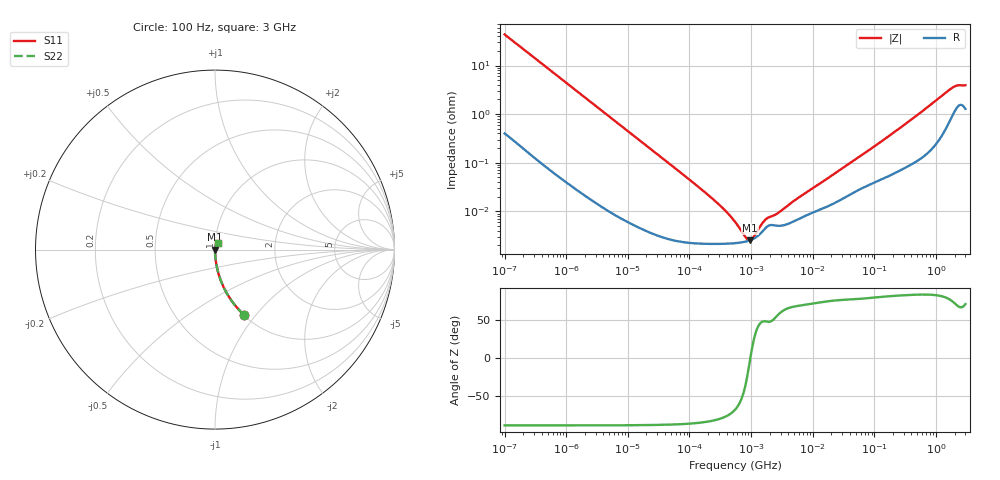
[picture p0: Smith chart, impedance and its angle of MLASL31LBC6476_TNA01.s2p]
! MLASL31LBC6476_TNA01  S-PARAMETER MODEL  ( Standard Model )
! Model Generated by TAIYO YUDEN Corporation (http://www.ty-top.com)
! Version 1.0
! TAIYO YUDEN Control No. 220601
! Copyright(c) 2018 TAIYO YUDEN CO.,LTD. All Rights Reserved.
! Product Description (link to TY-COMPAS)
! https://ds.yuden.co.jp/TYCOMPAS/or/detail?pn=MLASL31LBC6476MTNA01&u=M
! Products Name : Multilayer Ceramic Capacitors
! Characteristics :
!  Capacitance : 47 [uF] , Rated Voltage : 10 [V] , TCC : X6S
!  Case Size : 3.2 x 1.6 / 0.126 x 0.063 [mm/inch] , Thickness : 1.6 / 0.063 [mm/inch]
!  (Conditions: Temperature = 25 [degC] , DC Bias Voltage = 0 [V])
! External Node Assignments :
!  1  o---| |---o  2
! GND o---------o GND
! Frequency Range : 100Hz  -  3GHz  [ 401 STEP ]
# MHZ S RI R 50
! Freq[MHz].  S11 Real  S11 Imag  S21 Real  S21 Imag  S12 Real  S12 Imag  S22 Real  S22 Imag
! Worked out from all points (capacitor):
!   401 points, 100 Hz to 3 GHz, reference 50 ohm
!   read as one part in series: C = 36.5 uF near 109 Hz
!   lowest |Z| = 2.54 mohm at 958.4 kHz (marker M1)
!   series resonance near 973.7 kHz, so ESL is about 730 pH
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0.0001  0.1616 -0.3636  0.8384 0.3636  0.8384 0.3636  0.1616 -0.3636
0.000114  0.1302 -0.332  0.8698 0.332  0.8698 0.332  0.1302 -0.332
0.000175  0.0606 -0.2341  0.9394 0.2341  0.9394 0.2341  0.0606 -0.2341
0.000348  0.0167 -0.1237  0.9833 0.1237  0.9833 0.1237  0.0167 -0.1237
0.000724  0.00421 -0.0605  0.9958 0.0605  0.9958 0.0605  0.00421 -0.0605
0.001788  0.000844 -0.0247  0.9992 0.0247  0.9992 0.0247  0.000844 -0.0247
0.031977  3.28e-05 -0.00141  1 0.00141  1 0.00141  3.28e-05 -0.00141
0.16412  2.16e-05 -0.000268  1 0.000268  1 0.000268  2.16e-05 -0.000268
0.371814  2.15e-05 -0.000104  1 0.000104  1 0.000104  2.15e-05 -0.000104
0.423062  2.16e-05 -8.71e-05  1 8.71e-05  1 8.71e-05  2.16e-05 -8.71e-05
0.547723  2.21e-05 -5.69e-05  1 5.69e-05  1 5.69e-05  2.21e-05 -5.69e-05
0.958445  2.53e-05 -1.48e-06  1 1.48e-06  1 1.48e-06  2.53e-05 -1.48e-06
2.93481  5.03e-05 8.43e-05  0.9999 -8.43e-05  0.9999 -8.43e-05  5.03e-05 8.43e-05
3.198641  5.09e-05 9.4e-05  0.9999 -9.4e-05  0.9999 -9.4e-05  5.09e-05 9.4e-05
5.361412  6.54e-05 0.000163  0.9999 -0.000163  0.9999 -0.000163  6.54e-05 0.000163
9.794414  9.3e-05 0.000278  0.9999 -0.000278  0.9999 -0.000278  9.3e-05 0.000278
77.30952  0.000339 0.00169  0.9997 -0.00169  0.9997 -0.00169  0.000339 0.00169
175.1444  0.00055 0.00355  0.9994 -0.00355  0.9994 -0.00355  0.00055 0.00355
492.0662  0.00117 0.00938  0.9988 -0.00938  0.9988 -0.00938  0.00117 0.00938
1789.813  0.00955 0.0324  0.9904 -0.0324  0.9904 -0.0324  0.00955 0.0324
2219.584  0.015 0.0353  0.985 -0.0353  0.985 -0.0353  0.015 0.0353
3000  0.014 0.0362  0.986 -0.0362  0.986 -0.0362  0.014 0.0362
